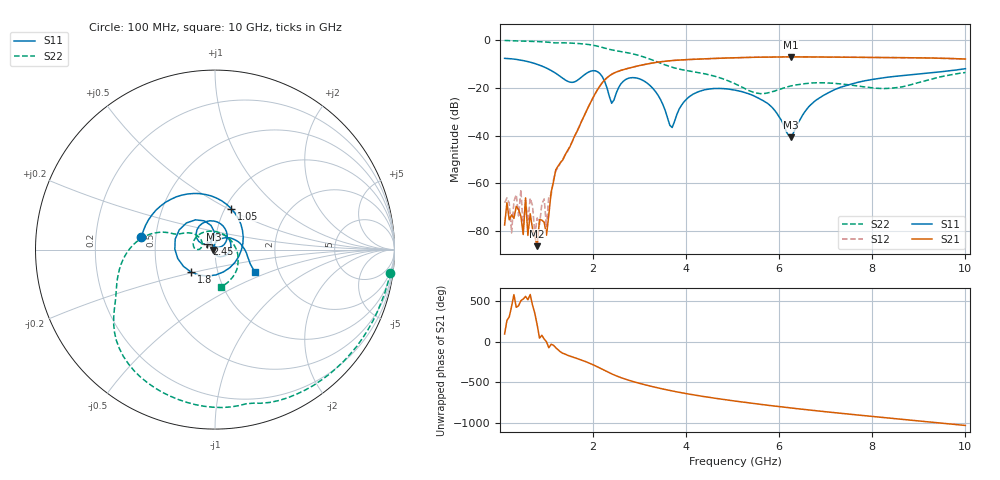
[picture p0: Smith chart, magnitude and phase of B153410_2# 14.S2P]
!  2-Port S-parameters saved by WinCal
! VAR MeasName=S-Parameters (CALIBRATED_DATA) read from VNA (N5245A)
! VAR MeasDate=2016-12-23 10:00:03
! VAR NAME=B153410_2# 14
! VAR FILENAME=B153410_2# 14.S2P
! VAR DATE=2016-12-23 10:00:03
! VAR PHYS_PORTS=1,2
# Hz S DB R 50
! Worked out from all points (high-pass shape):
!   199 points, 100 MHz to 10 GHz, reference 50 ohm
!   highest |S21| = -7.01 dB at 6.25 GHz (marker M1); lowest = -86.4 dB at 800 MHz (marker M2)
!   |S21| within 3 dB of the highest: 3.154 GHz to end of sweep
!   lowest |S11| = -40.7 dB at 6.25 GHz (marker M3), VSWR 1.02, Z = 49.1 + j0.0169 ohm
!   |S11| at or under -10 dB: 780.5 MHz to end of sweep
!   |S22| runs from -22.4 to -0.1 dB; largest |S21 - S12| = 0.0036
!   S11 on the Smith chart (normalised r, x): 100 MHz: 0.42, +0.07; 1.05 GHz: 1.07, +0.52; 1.8 GHz: 0.74, -0.19; 2.45 GHz: 0.91, +0.06; 10 GHz: 1.50, -0.39
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1e8  -7.62 170.4  -77.49 97.2  -68.16 103.2  -0.12 -7.5
2.5e8  -7.83 155.9  -73.26 79.0  -80.81 -2.8  -0.25 -17.7
4.5e8  -8.36 136.4  -73.83 149.6  -62.69 -2.3  -0.36 -30.9
5e8  -8.57 131.5  -81.47 170.1  -79.01 -141.4  -0.39 -34.2
5.5e8  -8.76 126.4  -66.16 -157.6  -66.96 -178.4  -0.42 -37.5
6e8  -8.99 121.2  -81.85 160.4  -76.09 -112.4  -0.45 -40.8
6.5e8  -9.24 116.1  -72.78 -134.6  -66.24 96.8  -0.49 -44.1
8e8  -10.13 99.8  -86.36 -150.8  -74.56 80.4  -0.59 -53.9
9.5e8  -11.25 81.9  -76.31 36.5  -66.57 21.4  -0.73 -63.7
1e9  -11.70 75.4  -81.76 1.0  -78.43 0.7  -0.79 -67.0
1.05e9  -12.20 68.5  -73.26 -72.3  -65.26 -17.5  -0.87 -70.3
1.2e9  -13.89 44.4  -54.30 -72.4  -54.66 -76.5  -1.15 -78.5
1.75e9  -15.53 -121.7  -34.16 135.3  -34.12 134.3  -1.51 -113.5
1.8e9  -14.74 -137.1  -32.06 124.7  -32.17 125.0  -1.60 -116.9
2.45e9  -25.06 147.3  -13.80 -48.0  -13.79 -47.9  -4.27 -154.6
3.4e9  -23.18 33.3  -9.20 150.5  -9.19 150.5  -9.28 164.2
3.7e9  -36.62 86.1  -8.56 113.5  -8.54 113.5  -11.34 159.9
5.05e9  -20.96 9.1  -7.37 -11.5  -7.37 -11.3  -18.27 141.8
6.25e9  -40.67 178.9  -7.01 -96.8  -7.02 -96.8  -19.18 178.1
6.7e9  -26.70 79.0  -7.03 -125.4  -7.05 -125.4  -17.96 163.9
8.35e9  -15.48 -1.4  -7.31 138.6  -7.29 139.0  -20.20 51.6
1e10  -11.96 -29.2  -7.92 46.9  -7.93 47.4  -13.56 -81.4
